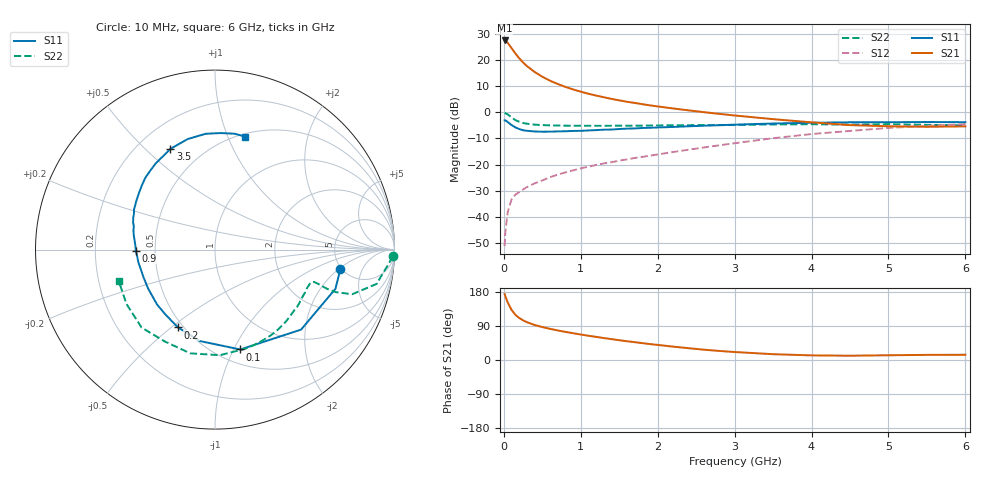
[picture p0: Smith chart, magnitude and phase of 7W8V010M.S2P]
! Infineon Technologies  Discrete & RF Semiconductors
! BFS17W
! Si NPN RF Bipolar Junction Transistor in SOT323
! VCE = 8 V  IC = 10 mA
! Common Emitter S-Parameters:  August  1999
# GHz  S  MA  R  50
!  f  S11  S21  S12  S22
! GHz  MAG  ANG  MAG  ANG  MAG  ANG  MAG  ANG
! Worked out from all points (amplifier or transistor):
!   36 points, 10 MHz to 6 GHz, reference 50 ohm
!   highest |S21| = 27.7 dB at 10 MHz (marker M1)
!   |S21| within 3 dB of that: start of sweep to 101.6 MHz
!   unconditionally stable (mu >= 1): 433 MHz to 2.184 GHz; 5.447 GHz to end of sweep
!   at 250 MHz: K = 0.78, MSG = 24.4 dB, |S12| = -29.6 dB
!   at 1.4 GHz: K = 1.17, MAG = 9.7 dB, |S12| = -19.1 dB
!   at 6 GHz: K = 1.04, MAG = -1.6 dB, |S12| = -4.5 dB
!   S11 on the Smith chart (normalised r, x): 10 MHz: 4.86, -2.13; 100 MHz: 0.64, -1.06; 200 MHz: 0.47, -0.53; 900 MHz: 0.39, -0.01; 3.5 GHz: 0.33, +0.60; 6 GHz: 0.53, +1.16
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0.01  0.7071 -8.9  24.18 174.1  0.0027 84.3  0.9912 -2.2
0.02  0.7057 -18.0  23.85 167.9  0.0051 85.5  0.9666 -5.2
0.05  0.6548 -42.9  21.77 151.9  0.0121 70.9  0.9201 -12.0
0.1  0.574 -75.8  17.25 132.4  0.0214 61.6  0.8042 -18.0
0.15  0.5164 -99.4  13.58 119.3  0.0264 55.4  0.7147 -19.4
0.2  0.4802 -115.4  11.01 110.8  0.0295 56.0  0.6631 -19.3
0.25  0.4551 -127.3  9.139 104.6  0.033 55.3  0.6281 -18.8
0.3  0.4449 -136.4  7.788 99.8  0.0369 56.9  0.609 -18.4
0.4  0.4312 -149.8  5.997 92.4  0.0434 59.0  0.5836 -18.1
0.5  0.4271 -158.5  4.856 86.9  0.0495 61.6  0.5724 -18.2
0.6  0.4276 -165.1  4.073 82.2  0.0569 62.8  0.5654 -19.0
0.7  0.4328 -170.6  3.525 78.0  0.064 64.6  0.5607 -20.1
0.9  0.4417 -179.3  2.77 70.7  0.0773 66.5  0.5553 -23.0
1.1  0.4516 173.2  2.291 63.9  0.091 67.8  0.5547 -26.7
1.3  0.4671 166.7  1.959 57.9  0.105 68.9  0.5541 -30.8
1.6  0.4893 158.6  1.607 49.5  0.1253 70.5  0.5563 -37.1
2.2  0.5271 143.7  1.194 35.3  0.1739 72.5  0.567 -51.7
2.8  0.5687 129.4  0.94 23.9  0.2337 71.8  0.5742 -67.7
3.5  0.6137 113.9  0.744 15.3  0.32 67.7  0.5891 -87.3
4.5  0.6474 94.6  0.572 11.3  0.442 55.9  0.5833 -118.7
5.5  0.6549 80.4  0.531 13.5  0.5532 42.6  0.5789 -148.4
6  0.6513 75.0  0.541 13.8  0.5972 36.0  0.5641 -161.7
